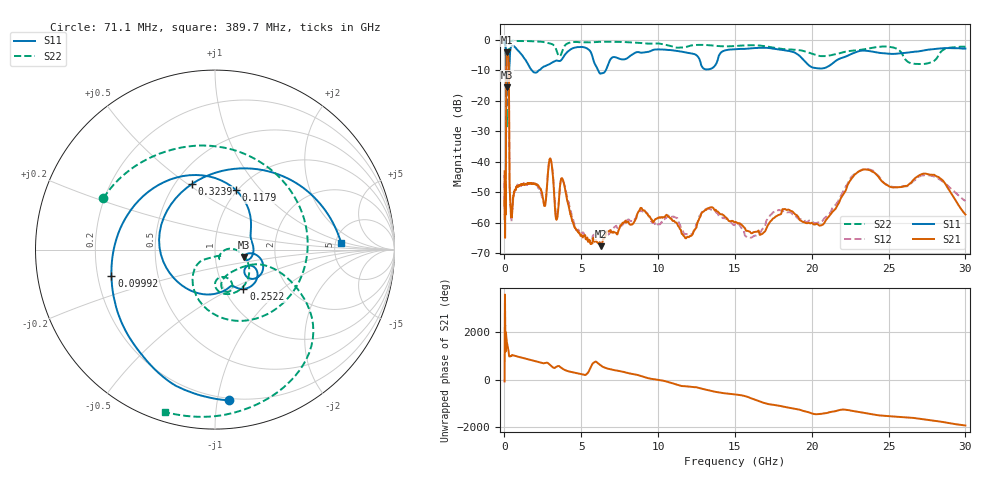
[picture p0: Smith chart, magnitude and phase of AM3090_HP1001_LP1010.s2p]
! Date/Time: Thu, Feb 28, 2019 2:03 PM
! Network Analyzer: Agilent Technologies E8364B Rev: A.07.50.67
! Sweep from 0.010 to 30.000 GHz, 1601 Points, Sweep Type: LOG
! Power Supply: 5.023 V, 0.002 A
# Hz S DB R 50
!freq MagS11 AngS11 MagS21 AngS21 MagS12 AngS12 MagS22 AngS22
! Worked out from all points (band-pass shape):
!   1601 points, 10 MHz to 30 GHz, reference 50 ohm
!   highest |S21| = -4.08 dB at 170.7 MHz (marker M1); lowest = -67.6 dB at 6.296 GHz (marker M2)
!   |S21| within 3 dB of the highest: 124.7 MHz to 273.7 MHz (149 MHz wide, 74.8 % of centre)
!   lowest |S11| = -15.6 dB at 154.4 MHz (marker M3), VSWR 1.40, Z = 68.9 - j6.01 ohm
!   |S11| at or under -10 dB: 119.6 MHz to 309.7 MHz (190.1 MHz wide, 88.6 % of centre); 1.794 GHz to 2.229 GHz (435 MHz wide, 21.6 % of centre); 6.098 GHz to 6.59 GHz (491.3 MHz wide, 7.75 % of centre)
!   |S22| runs from -28.5 to -0.2 dB; largest |S21 - S12| = 0.011
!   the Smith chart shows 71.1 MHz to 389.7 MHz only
!   S11 on the Smith chart (normalised r, x): 71.1 MHz: 0.19, -1.08; 99.92 MHz: 0.26, -0.12; 117.9 MHz: 0.98, +0.74; 252.2 MHz: 1.23, -0.58; 323.9 MHz: 0.60, +0.52; 389.7 MHz: 5.66, +0.78
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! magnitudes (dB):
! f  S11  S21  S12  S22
! 10 MHz  -0.2  -43.1  -48.7  -0.7
! 38.04 MHz  -0.5  -60.5  -57.9  -1.5
! 71.1 MHz  -1.5  -54.6  -51.4  -3.3
! 99.92 MHz  -4.5  -36.0  -35.7  -5.6
! 117.9 MHz  -9.1  -11.3  -11.3  -11.2
! 144.7 MHz  -14.2  -4.5  -4.5  -27.8
! 154.4 MHz  -15.6  -4.2  -4.2  -24.1
! 170.7 MHz  -12.6  -4.1  -4.1  -13.9
! 252.2 MHz  -11.4  -5.3  -5.3  -12.2
! 287.2 MHz  -12.0  -10.9  -10.9  -10.7
! 323.9 MHz  -8.2  -44.0  -43.6  -1.4
! 389.7 MHz  -3.0  -54.4  -53.6  -0.5
! 550.5 MHz  -1.9  -52.8  -53.6  -0.3
! 2.084 GHz  -10.7  -47.5  -47.4  -0.5
! 2.987 GHz  -7.7  -38.9  -39.0  -1.2
! 3.385 GHz  -6.7  -59.0  -57.6  -3.4
! 3.779 GHz  -6.1  -45.6  -45.5  -3.4
! 6.296 GHz  -10.9  -67.6  -63.6  -0.6
! 7.926 GHz  -6.2  -59.9  -60.3  -0.7
! 16.21 GHz  -2.7  -63.0  -64.4  -1.7
! 23.48 GHz  -3.5  -42.4  -42.3  -3.0
! 30 GHz  -2.8  -57.3  -52.8  -2.2
